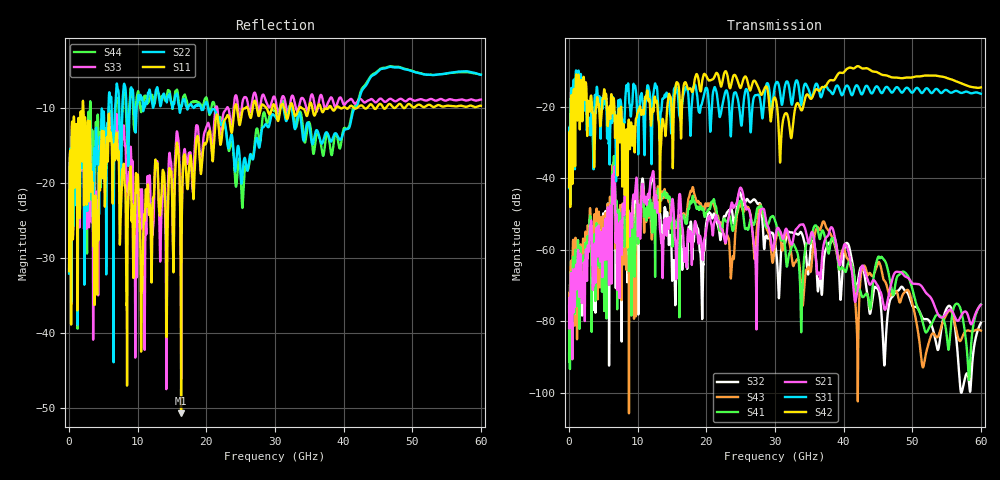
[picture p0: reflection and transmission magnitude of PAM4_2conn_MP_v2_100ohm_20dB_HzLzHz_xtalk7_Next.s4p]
! Info: Touchstone file created by Circ.  Input file=FAB50GbE_2conn_Midplane_Examax_Topo2_v2_100ohm_20dB_HzLzHz.circ
# Hz S RI R 50
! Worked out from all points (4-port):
!   6000 points, 10 MHz to 60 GHz, reference 50 ohm
!   strongest paths, dB at 10 MHz, 15.01 GHz, 30.01 GHz, 45.01 GHz, 60 GHz:
!     S42: -42.5, -25.2, -17.5, -10.5, -14.7
!     S31: -42.8, -20.4, -14.1, -14.6, -16.4
!     S21: -75.8, -46.1, -56.8, -70.1, -75.4
!     S41: -89.0, -56.5, -51.9, -62.1, -75.3
!     S43: -77.4, -52.6, -58.7, -63.6, -82.6
!     S32: -81.8, -68.3, -58.1, -71.0, -80.4
!   lowest |S11| = -50.8 dB at 16.32 GHz (marker M1), VSWR 1.01, Z = 49.7 - j0.0865 ohm
!   |S11| at or under -10 dB: start of sweep to 1.974 GHz; 2.079 GHz to 24.11 GHz (22.03 GHz wide, 168 % of centre); 24.48 GHz to 25.72 GHz (1.24 GHz wide, 4.94 % of centre)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
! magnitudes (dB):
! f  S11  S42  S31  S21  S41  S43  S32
! 10 MHz  -31.8  -42.5  -42.8  -75.8  -89.0  -77.4  -81.8
! 1.2 GHz  -37.0  -23.1  -20.7  -69.9  -68.4  -66.1  -74.5
! 6.4 GHz  -21.1  -18.5  -17.4  -40.9  -41.0  -39.5  -39.6
! 16.32 GHz  -50.8  -28.9  -21.7  -49.3  -50.7  -50.8  -57.3
! 24.9 GHz  -12.2  -14.7  -22.0  -42.8  -46.5  -47.5  -44.0
! 27.17 GHz  -9.2  -13.1  -16.8  -63.7  -51.2  -59.8  -46.2
! 60 GHz  -9.7  -14.7  -16.4  -75.4  -75.3  -82.6  -80.4
